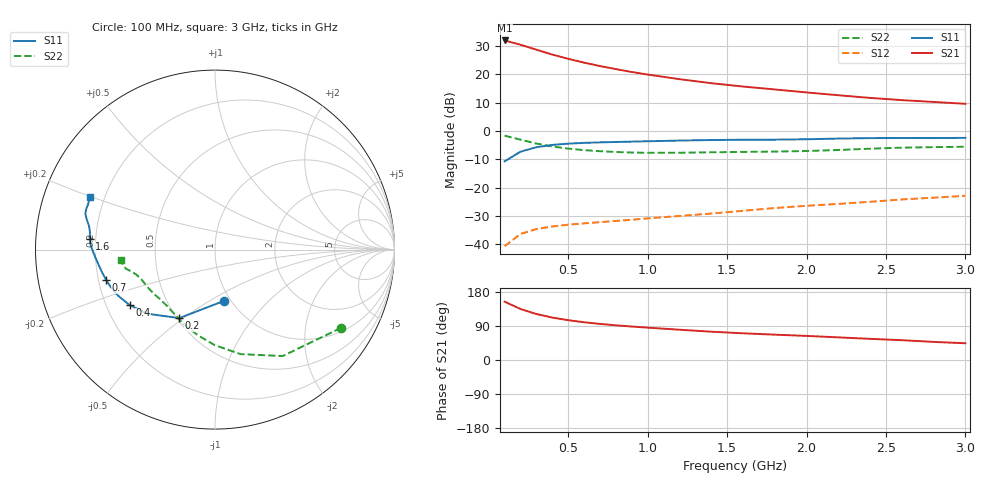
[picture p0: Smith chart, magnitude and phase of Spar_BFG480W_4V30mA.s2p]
! Filename: 430BFG480.001
! Title: BFG480W
! Bias: Vce=4V; Ic=30mA
! Company: NXP Semiconductors NL
! User: Quality&Reliability T&D
! Measure time: 10 Nov 1999 / 12:02:36
#  MHz  S  MA  R 50
! Freq  S11  S21  S12  S22  :
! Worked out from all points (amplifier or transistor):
!   20 points, 100 MHz to 3 GHz, reference 50 ohm
!   highest |S21| = 32.0 dB at 100 MHz (marker M1)
!   |S21| within 3 dB of that: start of sweep to 284.7 MHz
!   unconditionally stable (mu >= 1): 1.164 GHz to end of sweep
!   at 400 MHz: K = 0.51, MSG = 30.4 dB, |S12| = -33.8 dB
!   at 1.2 GHz: K = 1.01, MAG = 23.5 dB, |S12| = -30.0 dB
!   at 3 GHz: K = 1.08, MAG = 14.6 dB, |S12| = -22.9 dB
!   S11 on the Smith chart (normalised r, x): 100 MHz: 0.93, -0.58; 200 MHz: 0.51, -0.48; 400 MHz: 0.30, -0.27; 700 MHz: 0.23, -0.13; 1.6 GHz: 0.18, +0.04; 3 GHz: 0.14, +0.20
100  0.2906 -80.4  39.93 153.9  0.009196 63.7  0.8267 -31.8
200  0.4306 -117.6  33.56 134.6  0.01512 54.0  0.7027 -57.5
300  0.5176 -136.3  27.41 121.3  0.01845 48.2  0.5995 -76.3
400  0.5672 -146.9  22.49 112.0  0.02049 45.9  0.5321 -90.2
500  0.5981 -154.6  18.93 105.1  0.02204 45.4  0.4882 -100.9
600  0.6168 -160.1  16.19 99.6  0.02326 45.9  0.4593 -109.3
700  0.6297 -164.4  14.09 95.3  0.02444 47.4  0.4395 -116.0
800  0.6397 -168.0  12.43 91.5  0.02568 49.2  0.4255 -121.6
900  0.6492 -171.1  11.06 88.3  0.02699 51.5  0.4165 -126.6
1000  0.6588 -173.9  9.97 85.4  0.02847 53.4  0.4119 -131.0
1200  0.6776 -178.5  8.261 79.9  0.03148 57.0  0.4129 -138.6
1400  0.6925 178.2  7.014 74.7  0.03472 60.1  0.4205 -144.4
1600  0.7008 175.2  6.117 70.5  0.03879 63.1  0.4267 -148.8
1800  0.7033 172.1  5.434 66.9  0.04346 65.6  0.4332 -153.2
2000  0.7145 169.3  4.809 63.6  0.04757 67.6  0.4428 -158.2
2200  0.7348 166.7  4.293 59.7  0.05143 69.0  0.4616 -162.7
2400  0.7492 164.5  3.85 55.8  0.05596 69.6  0.4869 -165.9
2600  0.7523 162.6  3.517 52.3  0.06161 70.0  0.5079 -167.9
2800  0.7507 160.2  3.265 47.8  0.06624 69.4  0.5185 -170.2
3000  0.7562 157.4  3.029 44.2  0.07144 69.3  0.5268 -173.4
